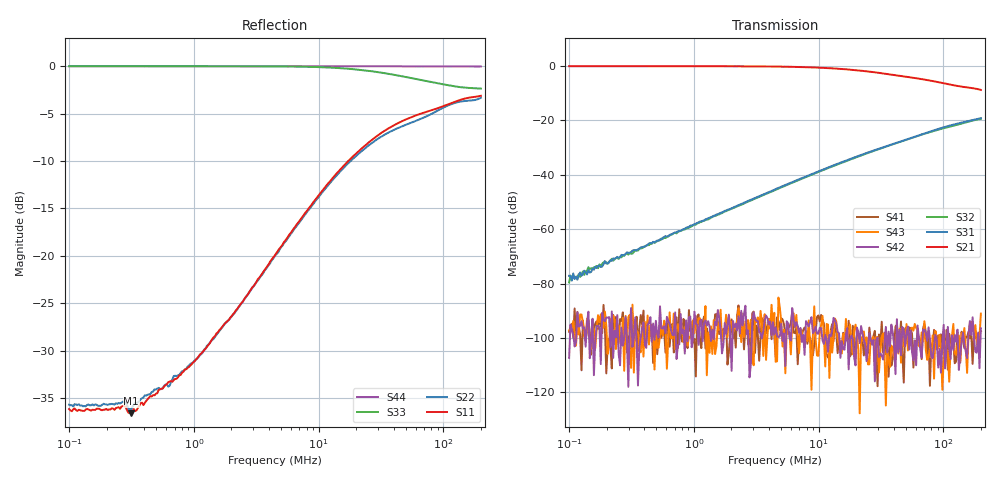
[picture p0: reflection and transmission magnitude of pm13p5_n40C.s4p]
!Keysight Technologies,E5080A,MY55200740,A.12.60.03
!Date: Friday, October 02, 2020 16:29:38
!Correction: S11(Full 4 Port(1,2,3,4))
!S12(Full 4 Port(1,2,3,4))
!S13(Full 4 Port(1,2,3,4))
!S14(Full 4 Port(1,2,3,4))
!S21(Full 4 Port(1,2,3,4))
!S22(Full 4 Port(1,2,3,4))
!S23(Full 4 Port(1,2,3,4))
!S24(Full 4 Port(1,2,3,4))
!S31(Full 4 Port(1,2,3,4))
!S32(Full 4 Port(1,2,3,4))
!S33(Full 4 Port(1,2,3,4))
!S34(Full 4 Port(1,2,3,4))
!S41(Full 4 Port(1,2,3,4))
!S42(Full 4 Port(1,2,3,4))
!S43(Full 4 Port(1,2,3,4))
!S44(Full 4 Port(1,2,3,4))
!S4P File: Measurements: <S11,S12,S13,S14>,
!<S21,S22,S23,S24>,
!<S31,S32,S33,S34>,
!<S41,S42,S43,S44>:Log Frequency Sweep
# Hz S  dB  R 50
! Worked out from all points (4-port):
!   300 points, 100 kHz to 200 MHz, reference 50 ohm
!   strongest paths, dB at 100 kHz, 673 kHz, 4.529 MHz, 30.48 MHz, 200 MHz:
!     S21: -0.1, -0.1, -0.3, -2.6, -8.9
!     S31: -77.1, -61.8, -45.3, -30.5, -19.2
!     S32: -79.6, -61.9, -45.6, -30.6, -19.5
!     S42: -107.3, -98.8, -96.1, -107.0, -96.4
!     S43: -97.2, -100.1, -108.7, -112.7, -91.0
!     S41: -97.7, -94.8, -106.9, -98.7, -97.6
!   lowest |S11| = -36.6 dB at 313.9 kHz (marker M1), VSWR 1.03, Z = 51.4 - j0.416 ohm
!   |S11| at or under -10 dB: start of sweep to 17.27 MHz
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100000  -36.16 0.8  -0.14 -0.1  -79.08 95.4  -88.15 106.0
        -0.14 -0.1  -35.69 1.3  -77.43 87.8  -100.42 -8.8
        -77.15 85.5  -79.58 85.5  0.00 -0.1  -122.76 -151.0
        -97.71 -125.5  -107.30 29.9  -97.22 -15.4  -0.00 -0.0
116477.3  -36.36 -2.1  -0.14 -0.2  -77.44 91.8  -96.86 168.5
          -0.14 -0.1  -35.74 -1.7  -77.64 92.2  -96.60 121.1
          -78.60 85.3  -77.39 87.8  0.00 -0.1  -96.99 -42.0
          -90.40 169.3  -90.54 36.4  -94.56 -61.9  0.00 -0.0
313913.9  -36.61 -15.9  -0.14 -0.4  -68.51 92.8  -99.49 23.9
          -0.14 -0.4  -36.19 -15.0  -68.39 91.9  -96.17 12.1
          -68.39 89.3  -69.02 89.4  -0.00 -0.4  -97.06 124.5
          -96.53 -23.0  -89.01 158.0  -110.98 56.2  -0.00 -0.0
4415652  -20.03 -91.9  -0.27 -5.2  -45.53 85.1  -93.32 122.0
         -0.27 -5.3  -20.11 -89.5  -45.76 85.5  -94.73 18.3
         -45.54 85.3  -45.76 85.7  -0.01 -5.3  -93.52 161.2
         -98.97 82.7  -98.67 -68.6  -90.74 54.0  -0.01 -0.3
2.13545e7  -8.85 -126.0  -1.74 -17.5  -32.96 72.7  -99.73 -18.8
           -1.75 -17.5  -9.13 -115.3  -33.17 75.7  -112.42 -53.2
           -32.94 72.6  -33.14 75.7  -0.38 -24.4  -107.19 -57.5
           -99.36 -143.6  -101.85 60.7  -127.65 -108.8  -0.00 -1.5
8.215269e7  -4.60 -154.2  -5.60 -21.9  -23.86 57.0  -98.52 -120.1
            -5.60 -21.9  -4.96 -132.7  -24.05 65.3  -95.37 151.1
            -23.85 57.0  -24.04 65.3  -1.71 -72.0  -106.63 46.2
            -103.19 68.5  -107.41 -177.7  -99.01 69.6  -0.01 -5.6
2e8  -3.12 -165.5  -8.86 -10.6  -19.24 36.4  -99.87 107.4
     -8.86 -10.6  -3.33 -113.1  -19.52 59.3  -97.10 81.5
     -19.23 36.4  -19.51 59.4  -2.36 -117.1  -89.95 -80.6
     -97.59 -149.3  -96.45 132.3  -91.03 -71.6  -0.03 -13.7
